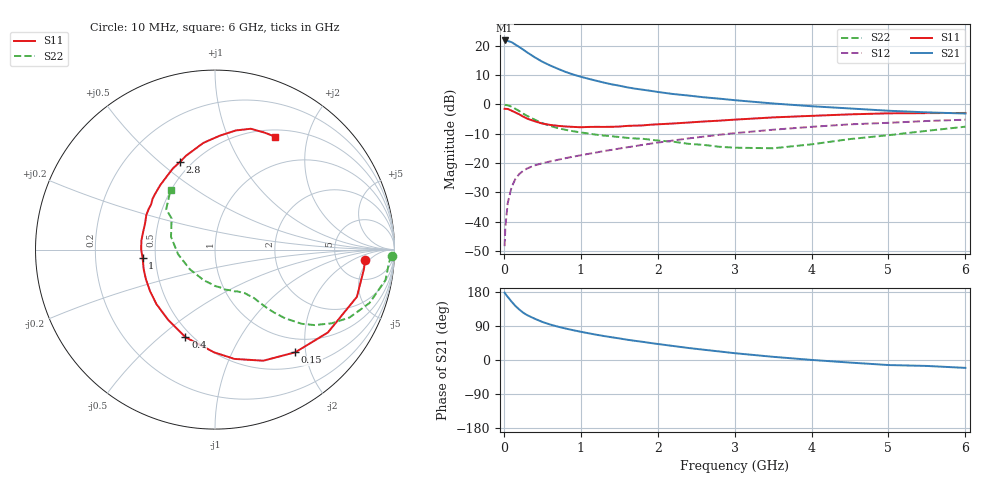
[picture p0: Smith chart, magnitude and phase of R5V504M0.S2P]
! SIEMENS Small Signal Semiconductors
! BFR183
! Si NPN RF Bipolar Junction Transistor in SOT23
! VCE = 0.5 V  IC = 4 mA
! Common Emitter S-Parameters:  May  1996
# GHz  S  MA  R  50
!  f  S11  S21  S12  S22
! GHz  MAG  ANG  MAG  ANG  MAG  ANG  MAG  ANG
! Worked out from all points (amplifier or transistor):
!   36 points, 10 MHz to 6 GHz, reference 50 ohm
!   highest |S21| = 21.8 dB at 10 MHz (marker M1)
!   |S21| within 3 dB of that: start of sweep to 244.5 MHz
!   unconditionally stable (mu >= 1): 1.003 GHz to 3.487 GHz
!   at 250 MHz: K = 0.38, MSG = 20.7 dB, |S12| = -22.7 dB
!   at 1.4 GHz: K = 1.10, MAG = 9.2 dB, |S12| = -15.5 dB
!   at 6 GHz: K = 0.98, MSG = 1.1 dB, |S12| = -5.2 dB
!   S11 on the Smith chart (normalised r, x): 10 MHz: 10, -4; 150 MHz: 0.75, -1.81; 400 MHz: 0.46, -0.61; 1 GHz: 0.42, -0.05; 2.8 GHz: 0.43, +0.59; 6 GHz: 0.59, +1.50
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0.01  0.8394 -3.9  12.3 177.6  0.0038 86.9  0.9848 -2.0
0.02  0.8366 -7.6  12.23 174.5  0.0081 88.3  0.9726 -4.1
0.05  0.8333 -18.4  12.05 166.6  0.0205 80.4  0.9651 -10.1
0.1  0.7803 -36.3  11.51 154.2  0.0384 71.4  0.9106 -19.1
0.15  0.7262 -52.0  10.46 142.6  0.0532 64.0  0.8394 -26.8
0.2  0.6751 -66.5  9.528 133.4  0.0647 58.6  0.7687 -32.3
0.25  0.6187 -79.9  8.61 125.1  0.0731 54.2  0.6955 -37.2
0.3  0.5725 -90.5  7.743 118.7  0.0801 51.2  0.6367 -40.5
0.4  0.5149 -108.7  6.365 109.1  0.0909 47.7  0.5476 -44.4
0.5  0.4701 -123.8  5.333 100.5  0.0987 46.1  0.4785 -46.9
0.6  0.4458 -137.0  4.617 93.8  0.1059 45.5  0.4288 -48.5
0.7  0.4298 -147.3  4.055 88.1  0.1129 45.6  0.3939 -49.6
0.8  0.419 -156.7  3.584 83.2  0.1204 45.8  0.3677 -50.4
1  0.406 -173.2  2.958 74.5  0.1351 46.4  0.3316 -52.0
1.1  0.4113 180.0  2.728 70.6  0.1429 46.9  0.3178 -53.5
1.6  0.4282 153.4  1.954 53.6  0.1848 47.6  0.2682 -60.9
2.2  0.4709 130.5  1.5 37.0  0.2413 45.3  0.2306 -75.4
2.8  0.5264 111.7  1.25 22.6  0.3024 40.4  0.1888 -99.5
3.5  0.5982 96.2  1.034 8.4  0.3688 32.1  0.178 -142.1
4.5  0.6742 80.0  0.85 -6.8  0.4557 19.3  0.2555 163.7
5.5  0.7077 67.2  0.729 -15.7  0.5198 7.8  0.3532 140.3
6  0.7129 62.0  0.697 -20.8  0.5467 0.1  0.4156 126.5
